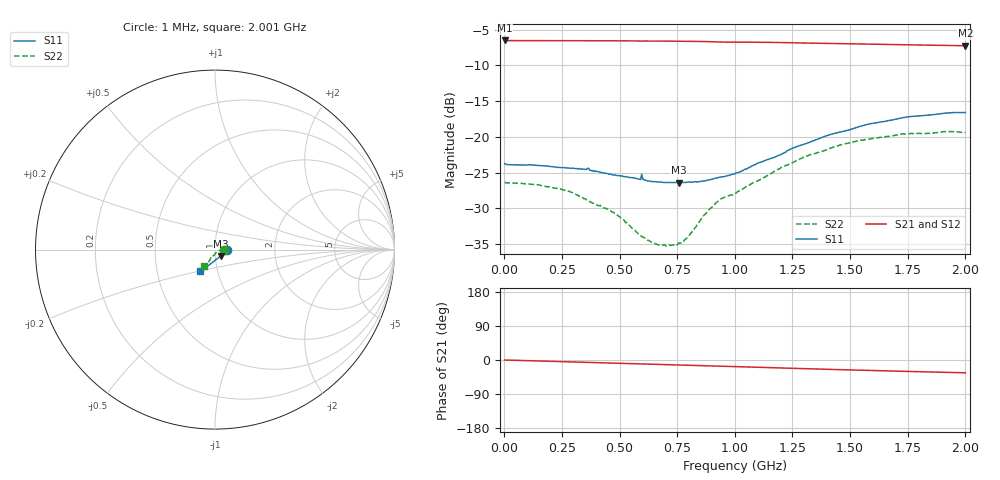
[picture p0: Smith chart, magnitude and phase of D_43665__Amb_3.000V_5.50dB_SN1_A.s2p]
! device id: 43665_
! dir: \\malibu\benchdata\1_engineers\tn_data\43665_75ohm\new\sparar\43665_\amb\3p000v\5p50db
! Serial: 1
! Insertion: A
! Temp: Amb
! VDD: 3.000V
! Attenuation Step: 5.50dB
! IDD: 1.453244e+00mA
! FILE NAME
! DATE 03-27-2009 08:34:43
! CORRECTED  DATA
#  Hz  S  RI  R  75
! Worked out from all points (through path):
!   401 points, 1 MHz to 2.001 GHz, reference 75 ohm
!   highest |S21| = -6.53 dB at 1 MHz (marker M1); lowest = -7.3 dB at 2.001 GHz (marker M2)
!   group delay of S21, straight-line fit = 47.8 ps
!   lowest |S11| = -26.4 dB at 756 MHz (marker M3), VSWR 1.10, Z = 79.7 - j5.72 ohm
!   |S11| at or under -10 dB: start of sweep to end of sweep
!   |S22| runs from -35.3 to -19.3 dB; largest |S21 - S12| = 0.0021
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1000000  0.0651 -0.00108  0.4717 -0.000794  0.4716 -0.000601  0.0483 -0.000574
1.56e8  0.063 -0.00432  0.4704 -0.0217  0.4706 -0.0217  0.0458 0.0022
2.76e8  0.06 -0.00931  0.4689 -0.0386  0.4691 -0.0385  0.0418 0.00265
3.36e8  0.0587 -0.0117  0.4677 -0.047  0.4679 -0.047  0.0379 0.00249
4.66e8  0.052 -0.0165  0.4648 -0.0652  0.4649 -0.0654  0.0298 -0.00121
5.11e8  0.0496 -0.0195  0.4634 -0.0718  0.4635 -0.0719  0.0266 -0.00297
5.91e8  0.044 -0.0241  0.4604 -0.0827  0.4604 -0.0829  0.0196 -0.00594
6.71e8  0.0385 -0.0294  0.4576 -0.0939  0.4576 -0.094  0.0139 -0.0108
7.11e8  0.0353 -0.0324  0.4559 -0.0997  0.4559 -0.0997  0.0111 -0.0135
7.56e8  0.0317 -0.0358  0.4538 -0.1062  0.4539 -0.1063  0.00727 -0.0166
7.96e8  0.0284 -0.039  0.4517 -0.112  0.4517 -0.1121  0.00354 -0.0197
8.66e8  0.0205 -0.0445  0.4473 -0.1223  0.4473 -0.1221  -0.00256 -0.0283
9.21e8  0.0142 -0.0496  0.4424 -0.1295  0.4426 -0.1293  -0.00852 -0.0338
9.51e8  0.0115 -0.0514  0.44 -0.1323  0.4402 -0.132  -0.0141 -0.035
1.001e9  0.00695 -0.0548  0.4382 -0.1371  0.4384 -0.1371  -0.0185 -0.0357
1.211e9  -0.018 -0.0747  0.4251 -0.1649  0.4257 -0.165  -0.0275 -0.0556
1.256e9  -0.0253 -0.0799  0.4212 -0.1703  0.4217 -0.1706  -0.0301 -0.0597
1.336e9  -0.0343 -0.0866  0.4151 -0.1791  0.4157 -0.1794  -0.0349 -0.0672
1.496e9  -0.0522 -0.0988  0.4016 -0.1965  0.4022 -0.1971  -0.0432 -0.0798
1.671e9  -0.0688 -0.1105  0.3872 -0.2137  0.387 -0.2147  -0.0502 -0.0877
1.916e9  -0.0841 -0.12  0.3668 -0.2345  0.3663 -0.2348  -0.0593 -0.0913
2.001e9  -0.0857 -0.1206  0.3601 -0.2411  0.3584 -0.2424  -0.0598 -0.0887
